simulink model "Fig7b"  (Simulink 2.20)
settings: Solver=ode45  StartTime=0.0  StopTime=10.0  RelTol=1e-3  AbsTol=1e-6
libraries: simulink x1

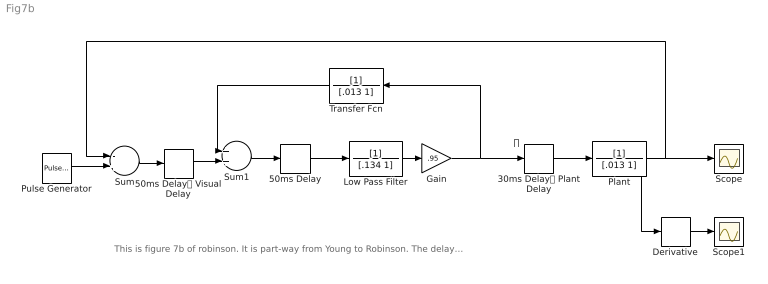
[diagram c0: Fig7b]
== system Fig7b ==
  note: 
  note: This is figure 7b of robinson. It is part-way from Young to Robinson. The delays have been parcelled out into their repective subsystems. Note that you do start to get significant oscillations in this model because the inner and outer feedback loops are now unmatched.
  30ms Delay Plant Delay : TransportDelay  DelayTime=.030  InitialInput=0  BufferSize=1024
  50ms Delay : TransportDelay  DelayTime=.050  InitialInput=0  BufferSize=1024
  50ms Delay Visual Delay : TransportDelay  DelayTime=.050  InitialInput=0  BufferSize=1024
  Derivative : Derivative
  Gain : Gain  Gain=.95
  Low Pass Filter : TransferFcn  Numerator=[1]  Denominator=[.134 1]
  Plant : TransferFcn  Numerator=[1]  Denominator=[.013 1]
  Pulse Generator : simulink/Sources/Pulse Generator  period=100  duty=50  amplitude=20  start=0
  Scope : Scope
  Scope1 : Scope
  Sum : Sum  Inputs=-+
  Sum1 : Sum  Inputs=++
  Transfer Fcn : TransferFcn  Orientation=left  Numerator=[1]  Denominator=[.013 1]
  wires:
  Plant/1 -> Scope/1, Sum/1, Derivative/1
  Pulse Generator/1 -> Sum/2
  Low Pass Filter/1 -> Gain/1
  50ms Delay/1 -> Low Pass Filter/1
  Sum1/1 -> 50ms Delay/1
  Transfer Fcn/1 -> Sum1/1
  Sum/1 -> 50ms Delay Visual Delay/1
  50ms Delay Visual Delay/1 -> Sum1/2
  Gain/1 -> 30ms Delay Plant Delay/1, Transfer Fcn/1
  30ms Delay Plant Delay/1 -> Plant/1
  Derivative/1 -> Scope1/1
